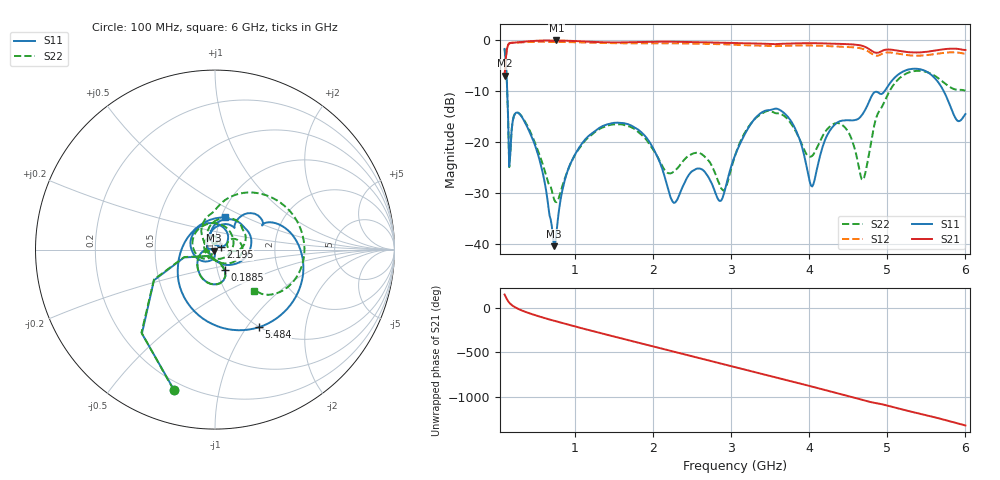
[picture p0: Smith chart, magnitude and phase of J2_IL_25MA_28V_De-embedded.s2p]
!Keysight Technologies,N5242B,MY61256241,Z.15.82.127
!Date: Friday, August 25, 2023 02:27:57
!Correction: S11(C  4-Port  )
!S31(C  4-Port  )
!S13(C  4-Port  )
!S33(C  4-Port  )
!S2P File: Measurements: S11, S31, S13, S33:
# Hz S  dB  R 50
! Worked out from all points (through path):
!   401 points, 100 MHz to 6 GHz, reference 50 ohm
!   highest |S21| = -0.11 dB at 763.8 MHz (marker M1); lowest = -7.0 dB at 100 MHz (marker M2)
!   group delay of S21, straight-line fit = 631 ps
!   lowest |S11| = -40.5 dB at 734.2 MHz (marker M3), VSWR 1.02, Z = 49.3 - j0.595 ohm
!   |S11| at or under -10 dB: 133.1 MHz to 4.968 GHz (4.835 GHz wide, 190 % of centre); 5.72 GHz to end of sweep
!   |S22| runs from -31.9 to -1.8 dB; largest |S21 - S12| = 0.065
!   S11 on the Smith chart (normalised r, x): 100 MHz: 0.16, -0.74; 188.5 MHz: 1.09, -0.25; 2.195 GHz: 1.06, +0.03; 5.484 GHz: 0.99, -1.14; 6 GHz: 1.04, +0.39
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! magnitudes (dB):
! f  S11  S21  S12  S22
! 100 MHz  -1.8  -7.0  -7.1  -1.8
! 159 MHz  -24.9  -0.7  -0.7  -25.0
! 188.5 MHz  -17.9  -0.6  -0.6  -17.9
! 262.2 MHz  -14.3  -0.5  -0.5  -14.2
! 439.2 MHz  -18.8  -0.2  -0.4  -18.4
! 734.2 MHz  -40.5  -0.1  -0.4  -31.3
! 763.8 MHz  -37.9  -0.1  -0.4  -31.9
! 881.8 MHz  -26.9  -0.2  -0.4  -26.7
! 1.088 GHz  -20.4  -0.3  -0.5  -20.6
! 1.649 GHz  -16.4  -0.5  -0.7  -16.8
! 2.076 GHz  -23.6  -0.3  -0.6  -23.5
! 2.195 GHz  -29.3  -0.3  -0.6  -26.2
! 2.593 GHz  -25.3  -0.5  -0.7  -22.2
! 2.858 GHz  -31.6  -0.5  -0.8  -28.6
! 3.05 GHz  -22.7  -0.6  -1.0  -22.8
! 3.611 GHz  -13.6  -0.8  -1.2  -14.4
! 4.038 GHz  -28.8  -0.6  -1.1  -22.8
! 4.392 GHz  -16.0  -0.8  -1.3  -16.4
! 4.687 GHz  -14.5  -1.2  -1.8  -27.5
! 5.027 GHz  -8.7  -1.9  -2.5  -10.1
! 5.484 GHz  -6.1  -2.4  -3.0  -6.2
! 6 GHz  -14.5  -2.0  -2.7  -9.9
